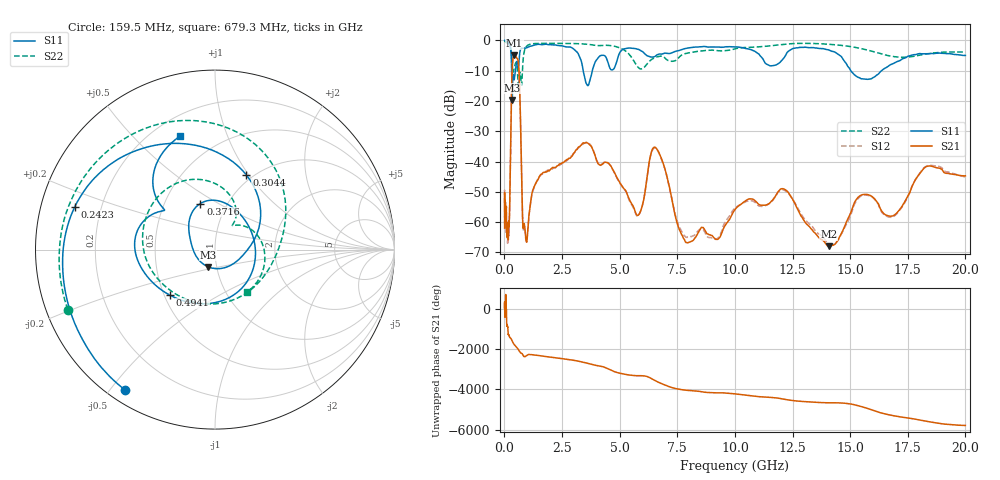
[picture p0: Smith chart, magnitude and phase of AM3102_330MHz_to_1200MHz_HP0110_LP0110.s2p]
! Date/Time: Tue, Sep 11, 2018 5:15 PM
! Network Analyzer: Agilent Technologies E8362B Rev: A.07.50.63
! Sweep from 0.010 to 20.000 GHz, 1601 Points, Sweep Type: LOG
! Power Supply: 4.949 V, 0.001 A
# Hz S DB R 50
!freq MagS11 AngS11 MagS21 AngS21 MagS12 AngS12 MagS22 AngS22
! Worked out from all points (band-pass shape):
!   1601 points, 10 MHz to 20 GHz, reference 50 ohm
!   highest |S21| = -4.90 dB at 438.8 MHz (marker M1); lowest = -67.9 dB at 14.07 GHz (marker M2)
!   |S21| within 3 dB of the highest: 348 MHz to 614.3 MHz (266.3 MHz wide, 55.3 % of centre)
!   lowest |S11| = -19.7 dB at 337.9 MHz (marker M3), VSWR 1.23, Z = 45.5 - j8.83 ohm
!   |S11| at or under -10 dB: 314.8 MHz to 478.4 MHz (163.6 MHz wide, 41.3 % of centre); 3.418 GHz to 3.815 GHz (396.4 MHz wide, 11 % of centre); 15.03 GHz to 16.37 GHz (1.341 GHz wide, 8.55 % of centre)
!   |S22| runs from -15.6 to -0.2 dB; largest |S21 - S12| = 0.0094
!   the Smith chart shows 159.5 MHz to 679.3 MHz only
!   S11 on the Smith chart (normalised r, x): 159.5 MHz: 0.05, -0.55; 242.3 MHz: 0.10, +0.15; 304.4 MHz: 0.93, +0.97; 371.6 MHz: 0.75, +0.42; 494.1 MHz: 0.53, -0.31; 679.3 MHz: 0.31, +0.69
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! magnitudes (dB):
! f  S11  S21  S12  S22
! 10 MHz  0.0  -62.0  -49.6  -0.2
! 35.55 MHz  0.0  -57.6  -58.7  -0.4
! 126.4 MHz  -0.4  -62.5  -62.9  -0.9
! 159.5 MHz  -0.6  -63.1  -61.6  -1.1
! 242.3 MHz  -1.8  -49.2  -49.4  -1.8
! 304.4 MHz  -6.9  -19.4  -19.4  -4.0
! 337.9 MHz  -19.7  -9.3  -9.4  -8.2
! 371.6 MHz  -11.4  -6.2  -6.3  -10.5
! 438.8 MHz  -12.4  -4.9  -4.9  -8.6
! 447.2 MHz  -11.9  -4.9  -4.9  -8.3
! 494.1 MHz  -8.9  -5.2  -5.3  -7.4
! 679.3 MHz  -3.6  -20.2  -20.2  -10.6
! 798.4 MHz  -2.6  -60.3  -60.7  -7.8
! 947.3 MHz  -2.5  -66.1  -66.3  -2.1
! 1.59 GHz  -1.4  -44.2  -44.3  -1.0
! 3.599 GHz  -14.8  -33.8  -33.7  -1.3
! 5.652 GHz  -2.7  -56.0  -56.3  -7.2
! 6.58 GHz  -5.0  -35.5  -35.7  -5.5
! 7.92 GHz  -2.6  -66.7  -65.0  -4.2
! 12.03 GHz  -6.6  -48.9  -49.2  -1.4
! 14.07 GHz  -3.2  -67.9  -67.1  -1.3
! 20 GHz  -5.0  -44.7  -45.1  -3.8
